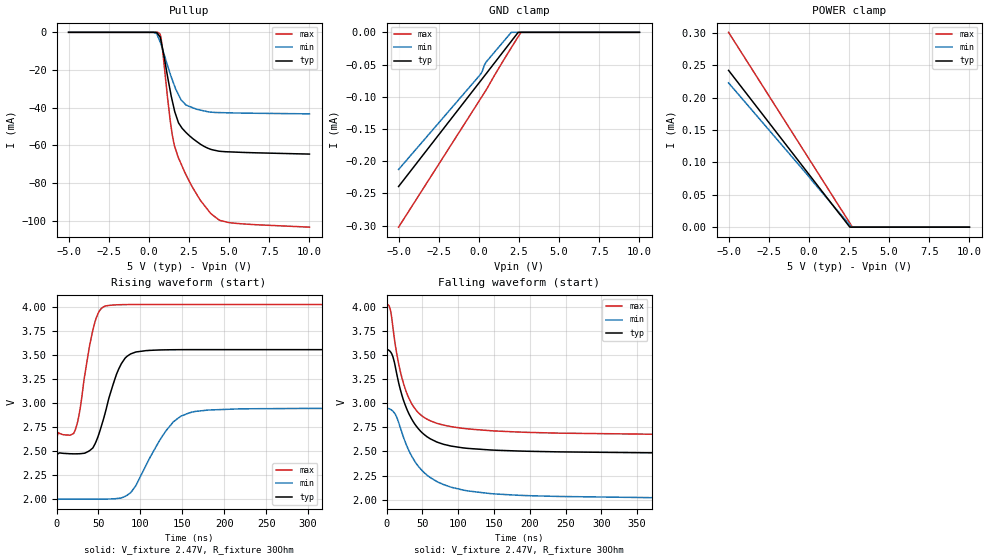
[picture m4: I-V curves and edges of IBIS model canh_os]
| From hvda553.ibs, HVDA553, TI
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|   canh_os Model
[Model]   canh_os
Model_type   I/O_open_source
Polarity   Inverting
Enable   Active-Low
Vinl = 0.5
Vinh = 0.9
Vmeas = 3.0
Vref = 2.47
Rref = 30
|   typ   min   max
|   (nom PVT)   (fast PVT)   (slow PVT)
C_comp   6.398e-12   6.051e-12   7.323e-12
| Where nom  PVT is Nominal Process, 5V, 27C
|   Fast PVT is Strong Process,  5.33V, -40C
|   Slow PVT is Weak Process,   4.68V, 150C
[Voltage Range]   5   4.68   5.33
|Junction Temperature
[Temperature Range]   27   150   -40
[Pullup Reference]   5   4.68   5.33
[Pulldown Reference]   0   0   0
[Power Clamp Reference]   5   4.68   5.33
[GND Clamp Reference]   0   0   0
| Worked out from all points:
|   slope of the pullup table from 0 to 0.75 V, typ, clamps not added: 175 ohm
|   falling waveform, V_fixture 2.47V, R_fixture 30Ohm: 20-80 % time 37ns typ, 50.6ns min, 30.9ns max; typ from 3.55 V to 2.47 V
|   rising waveform, V_fixture 2.47V, R_fixture 30Ohm: 20-80 % time 22.5ns typ, 37.4ns min, 15.2ns max; typ from 2.47 V to 3.55 V
[GND Clamp]
|   Voltage   I(typ)   I(min)   I(max)
-5V       -239.3uA   -212.9uA   -302.4uA
28.08mV   -77.9uA    -67.34uA   -106.1uA
196.6mV   -72.49uA   -61.14uA   -99.46uA
351mV     -67.53uA   -50.64uA   -93.41uA
454mV     -64.22uA   -46.23uA   -89.38uA
1.162V    -41.41uA   -25.17uA   -58.83uA
2.017V    -13.9uA    -47.64nA   -23.94uA
2.445V    -145.9nA   -26.5nA    -6.901uA
2.617V    0A         -17.99nA   -97.19nA
10V       0A         0A         0A
[Pullup]
|   Voltage   I(typ)   I(min)   I(max)
-5V       487.9nA    444.7nA    611.7nA
285.5mV   -3.049uA   -19.78uA   -6.367uA
491.4mV   -151.7uA   -781.6uA   -11.4uA
692.9mV   -2.388mA   -4.94mA    -881.7uA
836.8mV   -8.022mA   -8.642mA   -8.056mA
1.322V    -30.72mA   -21.98mA   -46.35mA
1.583V    -41.06mA   -28.15mA   -59.92mA
1.845V    -48.06mA   -33.15mA   -66.71mA
2.312V    -53.17mA   -38.62mA   -75.66mA
3.219V    -59.47mA   -41.32mA   -89.38mA
4.456V    -63.2mA    -42.64mA   -99.96mA
10V       -64.65mA   -43.3mA    -103.5mA
[POWER Clamp]
|   Voltage   I(typ)   I(min)   I(max)
-5V       242.1uA    222.8uA    300.9uA
2.55V     14.8nA     3.258uA    6.327uA
2.658V    0A         89.57nA    2.06uA
2.708V    0A         0A         113.2nA
10V       0A         0A         0A
[Ramp]
R_load = 30
|   typ   min   max
dV/dt_r   0.649218/2.24531e-08   0.565357/3.69359e-08   0.815694/1.51557e-08
dV/dt_f   0.647932/3.6995e-08   0.56377/5.05676e-08   0.814073/3.08604e-08
[Falling Waveform]
V_fixture = 2.47V
V_fixture_min = 2V
V_fixture_max = 2.66V
R_fixture = 30Ohm
|   Time   V(typ)   V(min)   V(max)
0s        3.553V     2.943V     4.022V
5.6ns     3.531V     2.935V     3.959V
9.2ns     3.474V     2.914V     3.769V
13.8ns    3.32V      2.862V     3.532V
21.4ns    3.084V     2.698V     3.265V
36.4ns    2.819V     2.435V     2.978V
61ns      2.631V     2.23V      2.818V
106ns     2.538V     2.101V     2.74V
372.8ns   2.485V     2.021V     2.678V
1.5us     2.473V     2.004V     2.665V
[Rising Waveform]
V_fixture = 2.47V
V_fixture_min = 2V
V_fixture_max = 2.66V
R_fixture = 30Ohm
|   Time   V(typ)   V(min)   V(max)
0s        2.471V     2.001V     2.662V
21.8ns    2.473V     2.002V     2.709V
26.6ns    2.473V     2.002V     2.864V
45.8ns    2.574V     2.002V     3.839V
64.2ns    3.101V     2.004V     4.014V
77ns      3.403V     2.014V     4.02V
88.6ns    3.51V      2.071V     4.021V
139.2ns   3.553V     2.803V     4.022V
181ns     3.554V     2.927V     4.022V
1.5us     3.553V     2.943V     4.022V
